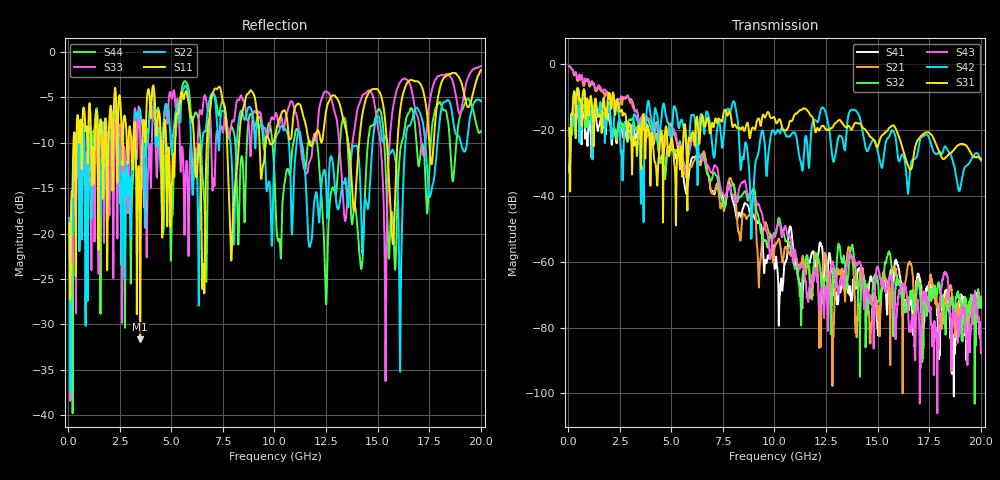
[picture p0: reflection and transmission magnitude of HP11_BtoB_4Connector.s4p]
# MHz S MA R 50.00
! FREQ  S11  S12  S13  S14
!  S21  S22  S23  S24
!  S31  S32  S33  S34
!  S41  S42  S43  S44
!  MAG  ANG  MAG  ANG  MAG  ANG  MAG  ANG
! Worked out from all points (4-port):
!   1996 points, 50 MHz to 20 GHz, reference 50 ohm
!   strongest paths, dB at 50 MHz, 5.04 GHz, 10.03 GHz, 15.02 GHz, 20 GHz:
!     S31: -19.5, -22.7, -16.9, -24.7, -28.7
!     S42: -19.5, -21.3, -21.2, -27.0, -29.3
!     S43: -0.6, -19.4, -52.0, -61.7, -87.7
!     S32: -32.8, -24.2, -51.4, -66.4, -74.0
!     S21: -0.6, -21.4, -55.1, -77.1, -73.0
!     S41: -32.3, -25.4, -61.1, -82.3, -73.3
!   lowest |S11| = -31.6 dB at 3.49 GHz (marker M1), VSWR 1.05, Z = 51.8 + j2.01 ohm
!   |S11| at or under -10 dB: 6.106 GHz to 6.723 GHz (616.9 MHz wide, 9.62 % of centre); 7.702 GHz to 8.279 GHz (577.5 MHz wide, 7.23 % of centre); 13.58 GHz to 14.1 GHz (524.4 MHz wide, 3.79 % of centre)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
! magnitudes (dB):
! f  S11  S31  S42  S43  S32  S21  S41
! 50 MHz  -18.9  -19.5  -19.5  -0.6  -32.8  -0.6  -32.3
! 3.49 GHz  -31.6  -20.0  -30.0  -17.2  -18.3  -18.0  -18.0
! 12.84 GHz  -4.8  -18.9  -29.4  -60.6  -62.4  -80.5  -65.9
! 13.6 GHz  -10.4  -18.7  -15.1  -57.6  -61.6  -55.4  -69.4
! 14.64 GHz  -4.3  -22.1  -24.5  -72.0  -71.2  -84.3  -64.6
! 15.38 GHz  -8.0  -20.6  -24.2  -69.0  -60.1  -65.6  -67.9
! 20 GHz  -2.0  -28.7  -29.3  -87.7  -74.0  -73.0  -73.3
